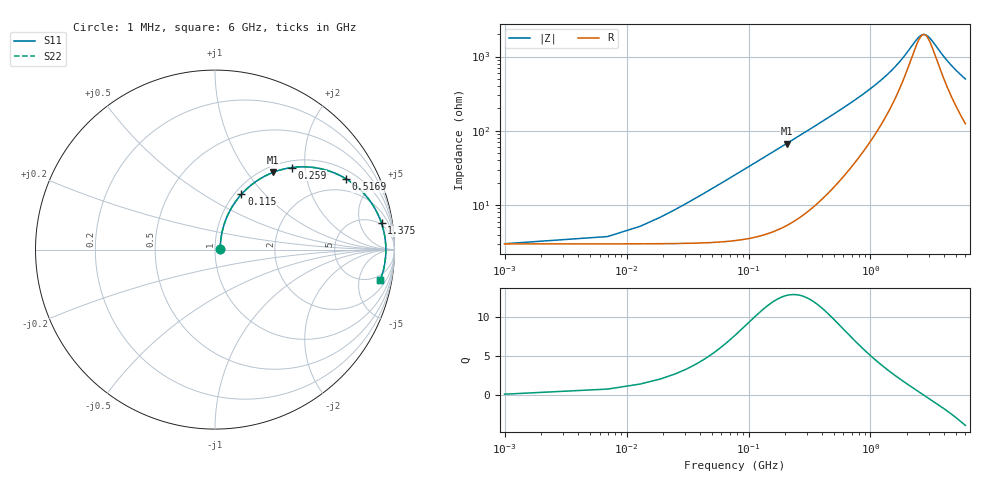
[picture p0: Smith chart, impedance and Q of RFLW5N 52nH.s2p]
!Vishay Electro-Films
!RFLW5N5200B - 52 nH Spiral Inductor on Quartz
!Measured in series configuration
!May 2011
# GHz S MA R 50
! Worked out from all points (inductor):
!   1001 points, 1 MHz to 6 GHz, reference 50 ohm
!   read as one part in series: L = 51.8 nH near 31 MHz
!   highest Q = 12.7 at 205 MHz (marker M1), where L = 52.1 nH
!   self-resonance near 2.738 GHz
!   S11 on the Smith chart (normalised r, x): 1 MHz: 1.06, +0.01; 115 MHz: 1.07, +0.75; 259 MHz: 1.13, +1.70; 516.9 MHz: 1.37, +3.46; 1.375 GHz: 4, +11; 6 GHz: 3, -10
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0.001  0.02926 6.0  0.9709 -0.2  0.9709 -0.2  0.02926 6.0
0.018997  0.0667 60.6  0.969 -3.4  0.969 -3.4  0.0667 60.6
0.042993  0.1379 69.8  0.9611 -7.7  0.9611 -7.7  0.1379 69.8
0.054991  0.1738 70.1  0.9551 -9.9  0.9551 -9.9  0.1738 70.1
0.078987  0.2438 68.6  0.939 -14.0  0.939 -14.0  0.2438 68.6
0.114981  0.3418 64.5  0.9067 -19.9  0.9067 -19.9  0.3418 64.5
0.156974  0.4426 59.0  0.8602 -26.2  0.8602 -26.2  0.4426 59.0
0.204966  0.5389 53.0  0.8011 -32.5  0.8011 -32.5  0.5389 53.0
0.258957  0.6249 47.0  0.7333 -38.5  0.7333 -38.5  0.6249 47.0
0.378937  0.7515 36.5  0.5973 -48.5  0.5973 -48.5  0.7515 36.5
0.516914  0.8303 28.3  0.4766 -55.7  0.4766 -55.7  0.8303 28.3
0.72088  0.8874 20.5  0.354 -61.5  0.354 -61.5  0.8874 20.5
1.00283  0.9213 14.1  0.2482 -64.6  0.2482 -64.6  0.9213 14.1
1.37477  0.9393 9.0  0.1637 -63.8  0.1637 -63.8  0.9393 9.0
2.00467  0.9496 3.9  0.08269 -50.5  0.08269 -50.5  0.9496 3.9
2.34061  0.9514 1.9  0.05856 -32.9  0.05856 -32.9  0.9514 1.9
2.56257  0.9519 0.8  0.05002 -15.5  0.05002 -15.5  0.9519 0.8
2.76654  0.952 -0.1  0.048 2.6  0.048 2.6  0.952 -0.1
3.0005  0.9519 -1.1  0.05173 21.1  0.05173 21.1  0.9519 -1.1
4.00233  0.949 -4.7  0.0953 55.3  0.0953 55.3  0.949 -4.7
5.00417  0.9435 -7.8  0.1432 62.9  0.1432 62.9  0.9435 -7.8
6  0.9365 -10.5  0.1877 65.1  0.1877 65.1  0.9365 -10.5
